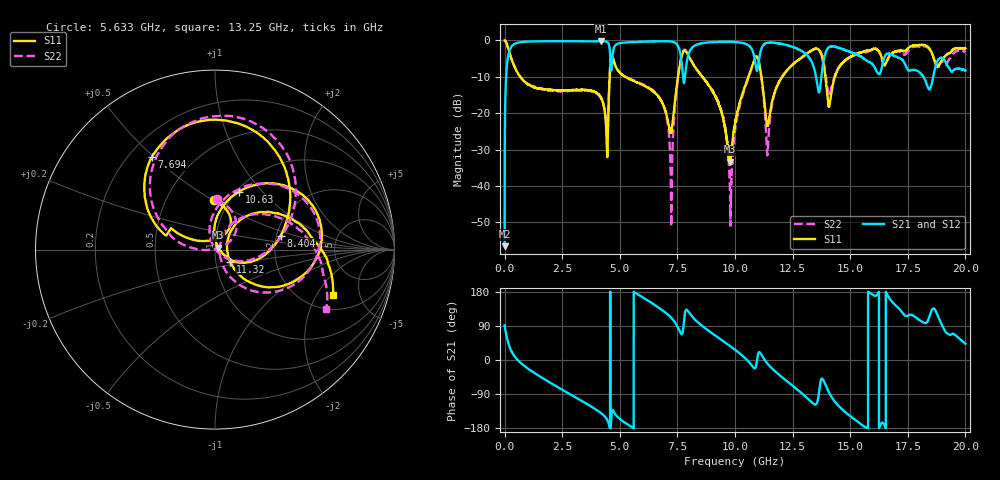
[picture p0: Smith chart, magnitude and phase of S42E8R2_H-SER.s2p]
! Created Wed Nov 25 21:51:10 2020
# khz S ma R 50
! 2 Port Network Data from SP1.SP block
! freq  magS11  angS11  magS21  angS21  magS12  angS12  magS22  angS22
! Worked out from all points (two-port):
!   20001 points, 300 kHz to 20 GHz, reference 50 ohm
!   highest |S21| = -0.20 dB at 4.184 GHz (marker M1); lowest = -56.5 dB at 300 kHz (marker M2)
!   |S21| within 3 dB of the highest: 192 MHz to 4.573 GHz (4.381 GHz wide, 184 % of centre); 4.704 GHz to 7.614 GHz (2.91 GHz wide, 47.3 % of centre)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
!   lowest |S11| = -33.3 dB at 9.777 GHz (marker M3), VSWR 1.04, Z = 51.9 + j1.18 ohm
!   |S11| at or under -10 dB: 678.9 MHz to 4.56 GHz (3.882 GHz wide, 148 % of centre); 5.246 GHz to 7.526 GHz (2.279 GHz wide, 35.7 % of centre); 8.58 GHz to 10.58 GHz (2.003 GHz wide, 20.9 % of centre)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
!   |S22| runs from -51.1 to 0.0 dB; largest |S21 - S12| = 0.019
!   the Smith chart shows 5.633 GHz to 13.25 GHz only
!   S11 on the Smith chart (normalised r, x): 5.633 GHz: 0.85, +0.51; 7.694 GHz: 0.29, +0.49; 8.404 GHz: 2.11, +0.38; 10.63 GHz: 1.03, +0.75; 11.32 GHz: 1.17, -0.16; 13.25 GHz: 2.80, -2.81
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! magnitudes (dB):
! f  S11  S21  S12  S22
! 300 kHz  0.0  -56.5  -56.5  0.0
! 110.3 MHz  -1.2  -6.2  -6.2  -1.2
! 291.3 MHz  -5.0  -1.8  -1.8  -4.9
! 3.334 GHz  -13.6  -0.2  -0.2  -13.7
! 4.184 GHz  -15.7  -0.2  -0.2  -15.8
! 4.681 GHz  -4.4  -4.4  -4.4  -4.2
! 5.633 GHz  -11.2  -0.4  -0.4  -11.1
! 6.667 GHz  -15.4  -0.2  -0.3  -15.2
! 7.233 GHz  -25.2  -0.3  -0.3  -51.1
! 7.694 GHz  -4.1  -6.7  -6.7  -3.8
! 8.404 GHz  -8.5  -1.0  -1.1  -8.5
! 9.389 GHz  -19.3  -0.4  -0.3  -18.8
! 9.777 GHz  -33.3  -0.4  -0.4  -40.3
! 10 GHz  -22.9  -0.4  -0.4  -24.8
! 10.63 GHz  -9.1  -1.6  -1.6  -9.4
! 11.01 GHz  -5.1  -7.0  -6.9  -5.3
! 11.32 GHz  -19.4  -0.8  -0.8  -21.8
! 13.25 GHz  -3.0  -5.0  -5.0  -3.1
! 13.33 GHz  -2.7  -6.0  -5.9  -2.7
! 14.09 GHz  -17.9  -1.8  -1.8  -15.0
! 16.67 GHz  -4.7  -3.6  -3.8  -4.7
! 20 GHz  -2.1  -8.3  -8.2  -3.3
